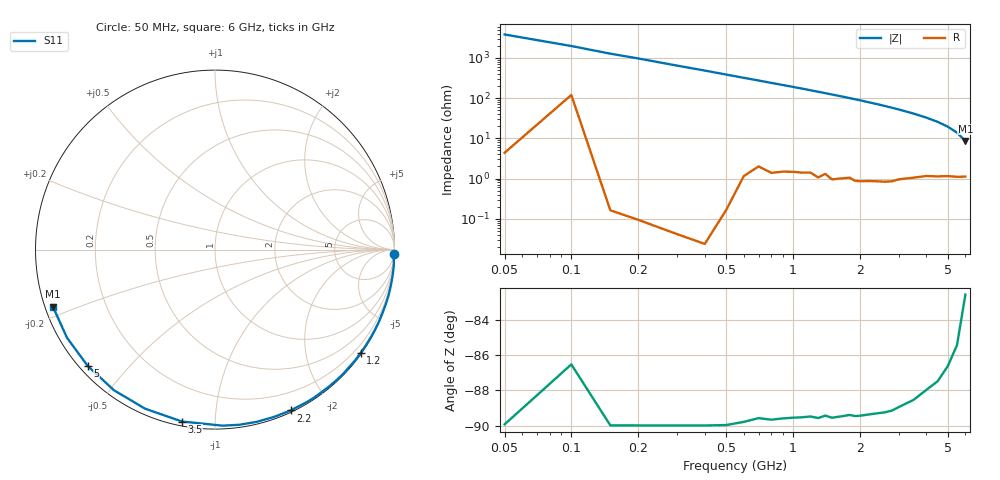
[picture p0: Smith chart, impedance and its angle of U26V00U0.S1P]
! SIEMENS Discrete & RF Semiconductors
! BBY52-02W
! Si Tuning Diode in SCD-80
! VR = 6 V
! S-Parameters:  September  1997
# GHz  S  MA  R  50
!  f  S11
! GHz  MAG  ANG
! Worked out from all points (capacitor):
!   34 points, 50 MHz to 6 GHz, reference 50 ohm
!   read as one part to ground: C = 833 fF near 50 MHz
!   lowest |Z| = 8.62 ohm at 6 GHz (marker M1)
!   S11 on the Smith chart (normalised r, x): 50 MHz: 0, -76; 1.2 GHz: 0.03, -3.13; 2.2 GHz: 0.02, -1.58; 3.5 GHz: 0.02, -0.83; 5 GHz: 0.02, -0.39; 6 GHz: 0.02, -0.17
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0.05  1 -1.5
0.1  0.9969 -2.9
0.15  1 -4.5
0.2  1 -5.9
0.4  1 -11.8
0.5  0.9999 -14.8
0.6  0.9989 -17.8
0.8  0.9977 -23.7
1  0.9962 -29.5
1.1  0.9956 -32.4
1.2  0.9948 -35.4
1.3  0.9954 -38.4
1.5  0.9946 -44.3
1.6  0.9937 -47.2
1.7  0.9927 -50.1
1.9  0.9922 -56.0
2  0.9918 -58.9
2.2  0.9901 -64.8
2.4  0.9887 -70.6
2.6  0.9873 -76.3
2.8  0.9854 -82.0
3  0.9819 -87.5
3.5  0.9753 -100.9
4  0.9681 -113.7
4.5  0.9649 -125.7
5  0.9608 -137.5
5.5  0.9598 -149.2
6  0.9575 -160.6
